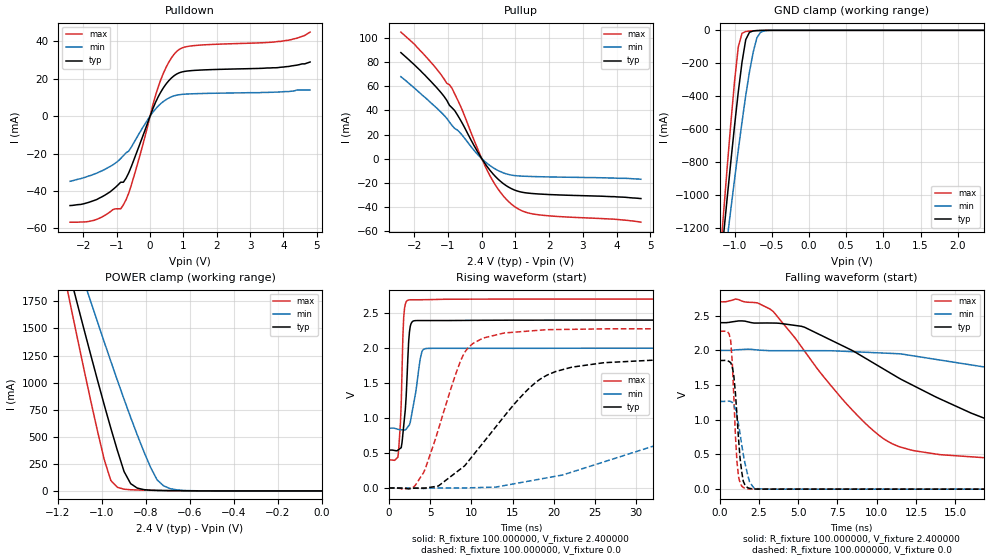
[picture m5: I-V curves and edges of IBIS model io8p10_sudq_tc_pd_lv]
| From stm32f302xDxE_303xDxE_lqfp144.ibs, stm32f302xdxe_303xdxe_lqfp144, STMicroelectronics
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|   Model io8p10_sudq_tc_pd_lv
[Model]  io8p10_sudq_tc_pd_lv
Model_type I/O
Polarity   Non-Inverting
Enable   Active-Low
Vinl =   0.720000V
Vinh =   1.680000V
Vmeas =  1.200000V
Cref =   50.000000pF
Rref =   100.000000M
Vref =   0.0V
C_comp   1.378000pF   1.292700pF   1.486400pF
[Temperature Range]   25.000000   0.125000k   -40.000000
[Pullup Reference]   2.400000V   2.000000V   2.700000V
[Pulldown Reference]   0.0V   0.0V   0.0V
[POWER Clamp Reference]   2.400000V   2.000000V   2.700000V
[GND Clamp Reference]   0.0V   0.0V   0.0V
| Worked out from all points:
|   slope of the pulldown table from 0 to 0.36 V, typ, clamps not added: 25.7 ohm
|   slope of the pullup table from 0 to 0.36 V, typ, clamps not added: 26.8 ohm
|   GND clamp passes 1 mA (typ) near -0.67 V on its own axis
|   POWER clamp passes 1 mA (typ) near -0.60 V on its own axis
|   rising waveform, R_fixture 100.000000, V_fixture 2.400000: 20-80 % time 554ps typ, 891ps min, 361ps max; typ from 0.541 V to 2.4 V
|   rising waveform, R_fixture 100.000000, V_fixture 0.0: 20-80 % time 8.01ns typ, 22.8ns min, 3.78ns max; typ from 0 V to 1.85 V
|   falling waveform, R_fixture 100.000000, V_fixture 2.400000: 20-80 % time 10.1ns typ, 24ns min, 5.13ns max; typ from 2.4 V to 0.541 V
|   falling waveform, R_fixture 100.000000, V_fixture 0.0: 20-80 % time 376ps typ, 593ps min, 283ps max; typ from 1.85 V to 0 V
[Pulldown]
|Voltage   I(typ)   I(min)   I(max)
-2.4V     -47.8mA    -34.8mA    -56.7mA
-1.68V    -45.1mA    -31mA      -55.7mA
-1.12V    -39.3mA    -26.1mA    -50.03mA
-800mV    -35.33mA   -21.13mA   -47.42mA
-640mV    -30.33mA   -18.65mA   -41.16mA
-480mV    -23.12mA   -14mA      -31.94mA
240mV     10.22mA    5.339mA    15.38mA
480mV     17.22mA    8.864mA    26.1mA
800mV     22.59mA    11.27mA    34.68mA
1.36V     24.54mA    12.05mA    37.84mA
3.92V     26.2mA     13mA       40mA
4.8V      29mA       14mA       45mA
[Pullup]
|Voltage   I(typ)   I(min)   I(max)
-2.4V     88mA       68mA       105mA
-2V       77.9mA     58.6mA     95mA
-1.36V    59.6mA     42.6mA     75.1mA
-880mV    42.13mA    27.44mA    58.22mA
-560mV    28.45mA    18.75mA    39mA
-160mV    7.44mA     4.66mA     10.64mA
160mV     -6.607mA   -3.947mA   -9.704mA
480mV     -16.91mA   -9.806mA   -25.1mA
880mV     -24.89mA   -13.63mA   -37.75mA
1.2V      -27.87mA   -14.5mA    -43.37mA
1.6V      -29.13mA   -14.89mA   -46.24mA
4.72V     -33.1mA    -17.1mA    -52.7mA
[GND_clamp]
|Voltage   I(typ)   I(min)   I(max)
-2.4V     -7.358A    -6.372A    -8.78A
-1.2V     -1.489A    -1.65A     -1.416A
-1.15V    -1.254A    -1.461A    -1.124A
-1.1V     -1.024A    -1.273A    -838.2mA
-1.05V    -797.6mA   -1.088A    -563.2mA
-950mV    -374.6mA   -728.7mA   -100.8mA
-900mV    -194.3mA   -558mA     -18.03mA
-850mV    -56.96mA   -397.5mA   -7.097mA
-750mV    -3.597mA   -133.8mA   -2.788mA
-700mV    -1.53mA    -44.71mA   -1.533mA
-600mV    -249.2uA   -2.951mA   -225.1uA
2.35V     60.02uA    46.69uA    67.1uA
[POWER_clamp]
|Voltage   I(typ)   I(min)   I(max)
-2.4V     9.979A     9.967A     9.901A
-1.17V    2.182A     2.481A     1.978A
-1.14V    1.945A     2.294A     1.683A
-1.11V    1.71A      2.108A     1.391A
-1.08V    1.476A     1.923A     1.102A
-1.05V    1.245A     1.739A     819.9mA
-960mV    578.2mA    1.196A     96.06mA
-900mV    179.5mA    846.7mA    16.04mA
-870mV    67.18mA    678.8mA    10.82mA
-780mV    6.749mA    219.9mA    5.853mA
-720mV    3.355mA    46.34mA    3.808mA
0V        0A         0A         0A
[Ramp]
| variable   typ   min   max
dV/dt_r  1.11246/8.00350n   0.75714/22.76270n   1.36494/3.77653n
dV/dt_f  1.11458/10.04491n   0.68704/24.05730n   1.37923/5.11829n
R_load = 100.000000
[Rising Waveform]
R_fixture= 100.000000
V_fixture= 2.400000
V_fixture_min= 2.000000
V_fixture_max= 2.700000
|time   V(typ)   V(min)   V(max)
0s        541.2mV    853.5mV    400.3mV
1.101ns   541.8mV    838.8mV    442.2mV
1.401ns   568.2mV    832.5mV    921.2mV
1.802ns   890.6mV    830.2mV    2.439V
2.102ns   1.315V     841.3mV    2.662V
2.302ns   1.854V     873.2mV    2.683V
2.703ns   2.351V     1.008V     2.689V
3.804ns   2.392V     1.844V     2.689V
4.404ns   2.392V     1.99V      2.69V
49.85ns   2.399V     1.999V     2.699V
[Rising Waveform]
R_fixture= 100.000000
V_fixture= 0.0
V_fixture_min= 0.0
V_fixture_max= 0.0
|time   V(typ)   V(min)   V(max)
0s        765pV      13.32nV    588.1pV
3.003ns   -3.008mV   -2.703mV   13.26mV
4.204ns   -806.8uV   -7.147mV   218.7mV
9.409ns   348.2mV    1.518mV    1.972V
14.01ns   1.028V     35.19mV    2.215V
19.22ns   1.614V     146.5mV    2.262V
26.23ns   1.791V     378.7mV    2.274V
43.04ns   1.847V     952.6mV    2.275V
55.06ns   1.855V     1.158V     2.275V
99.7ns    1.854V     1.264V     2.275V
[Falling Waveform]
R_fixture= 100.000000
V_fixture= 2.400000
V_fixture_min= 2.000000
V_fixture_max= 2.700000
|time   V(typ)   V(min)   V(max)
0s        2.399V     1.999V     2.699V
3.203ns   2.394V     1.995V     2.595V
5.405ns   2.333V     1.995V     1.989V
9.81ns    1.815V     1.967V     838.9mV
11.41ns   1.6V       1.951V     613.7mV
14.01ns   1.302V     1.861V     497.5mV
20.22ns   786.4mV    1.641V     430.2mV
27.63ns   612.4mV    1.382V     407.1mV
53.45ns   543.2mV    936.8mV    400.2mV
99.7ns    541.2mV    853.5mV    400.3mV
[Falling Waveform]
R_fixture= 100.000000
V_fixture= 0.0
V_fixture_min= 0.0
V_fixture_max= 0.0
|time   V(typ)   V(min)   V(max)
0s        1.854V     1.264V     2.275V
700.7ps   1.822V     1.263V     2.14V
900.9ps   1.631V     1.207V     1.326V
1.101ns   1.061V     1.061V     391.7mV
1.201ns   720.8mV    934.1mV    178.5mV
1.401ns   252.7mV    642.4mV    44.96mV
1.702ns   34.65mV    284.2mV    6.963mV
2.202ns   3.035mV    14.56mV    1.174mV
2.903ns   592.3uV    2.144mV    1.041mV
49.85ns   765pV      13.32nV    588.1pV
